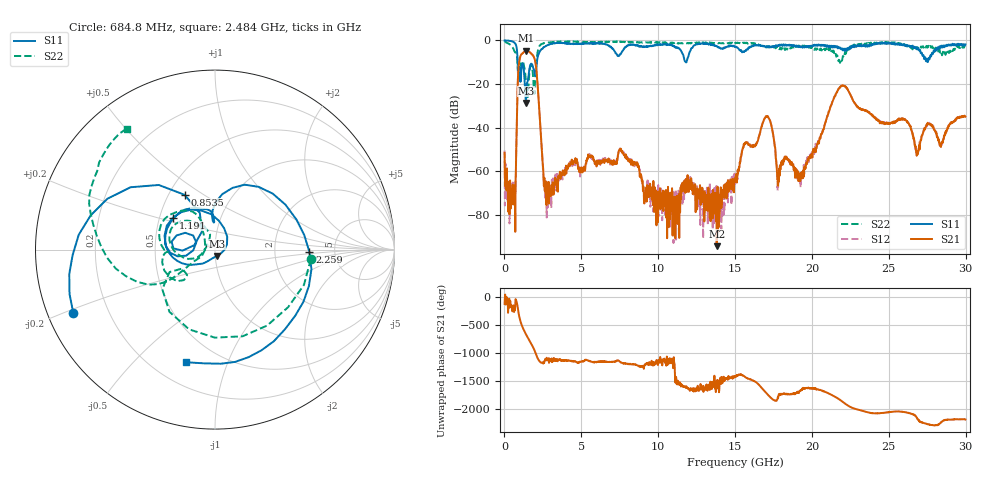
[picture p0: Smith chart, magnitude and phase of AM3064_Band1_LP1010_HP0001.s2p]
# Hz S DB R 50.0
!freq dBS11 angS11 dBS21 angS21 dBS12 angS12 dBS22 angS22
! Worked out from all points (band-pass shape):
!   1600 points, 10 MHz to 29.98 GHz, reference 50 ohm
!   highest |S21| = -4.73 dB at 1.416 GHz (marker M1); lowest = -94.5 dB at 13.81 GHz (marker M2)
!   |S21| within 3 dB of the highest: 1.019 GHz to 1.921 GHz (902.1 MHz wide, 61.4 % of centre)
!   lowest |S11| = -28.7 dB at 1.397 GHz (marker M3), VSWR 1.08, Z = 50.8 - j3.61 ohm
!   |S11| at or under -10 dB: 857.5 MHz to 2.111 GHz (1.254 GHz wide, 84.5 % of centre); 11.79756 GHz to 11.83685 GHz (39.28 MHz wide, 0.332 % of centre)
!   |S22| runs from -26.0 to -0.4 dB; largest |S21 - S12| = 0.0077
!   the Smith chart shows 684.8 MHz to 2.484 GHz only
!   S11 on the Smith chart (normalised r, x): 684.8 MHz: 0.08, -0.21; 853.5 MHz: 0.60, +0.42; 1.191 GHz: 0.59, +0.23; 2.259 GHz: 3.22, -0.13; 2.484 GHz: 0.33, -0.72
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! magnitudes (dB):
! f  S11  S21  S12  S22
! 10 MHz  0.0  -51.6  -50.6  -0.4
! 366.1 MHz  -0.2  -64.3  -66.1  -1.9
! 684.8 MHz  -1.3  -68.3  -67.9  -5.4
! 853.5 MHz  -9.1  -22.3  -22.2  -11.0
! 1.191 GHz  -10.6  -5.9  -5.8  -9.6
! 1.397 GHz  -28.7  -4.7  -4.7  -18.5
! 1.416 GHz  -25.8  -4.7  -4.7  -19.4
! 2.259 GHz  -5.6  -31.3  -31.2  -2.8
! 2.484 GHz  -3.8  -56.2  -55.1  -1.6
! 2.822 GHz  -2.1  -67.3  -77.3  -0.9
! 5.015 GHz  -1.4  -58.9  -60.1  -0.7
! 7.582 GHz  -6.0  -49.8  -50.6  -0.7
! 10 GHz  -2.0  -69.4  -66.5  -1.0
! 13.81 GHz  -2.6  -94.5  -68.1  -1.2
! 15 GHz  -2.9  -64.6  -65.9  -1.4
! 17.03 GHz  -3.0  -34.8  -34.9  -3.2
! 17.84 GHz  -2.4  -62.8  -65.0  -3.4
! 19.99 GHz  -2.8  -52.5  -51.6  -3.2
! 21.94 GHz  -4.1  -20.8  -20.8  -9.4
! 25 GHz  -1.1  -38.3  -37.8  -1.1
! 26.85 GHz  -4.2  -51.2  -52.3  -3.1
! 29.98 GHz  -1.9  -35.0  -34.8  -3.2
